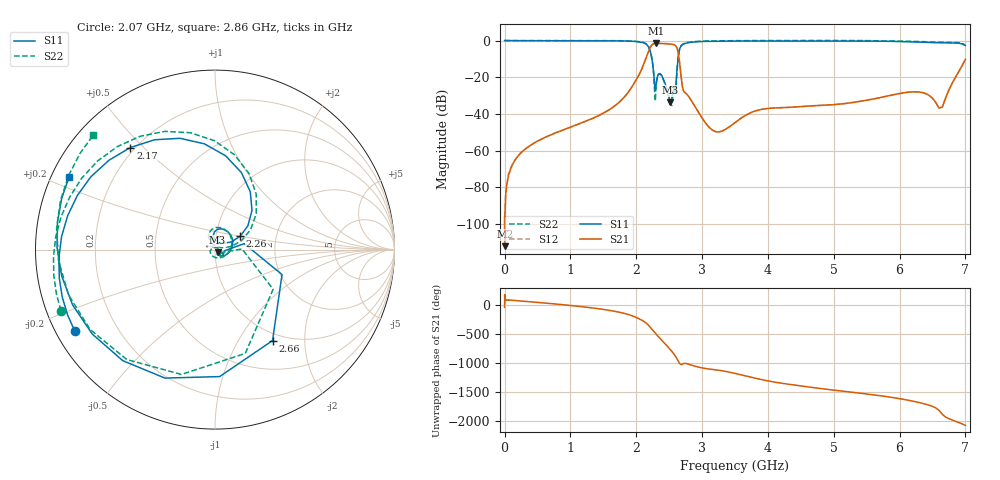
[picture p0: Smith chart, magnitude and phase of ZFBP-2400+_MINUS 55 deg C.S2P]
! Mini-Circuits
! S2P DATA File Format
! Type: BAND PASS FILTER
! Model: ZFBP-2400+
! All S Parameters are in dB deg format
! TEST CONDITIONS: INPUT POWER = 0 dBm @ Temperature = - 55 deg C
! 401 Frequency points
# MHz S DB R 50
!FREQMAG(S11)PHS(S11)MAG(S21)PHS(S21)MAG(S12)PHS(S12)MAG(S22)PHS(S22)
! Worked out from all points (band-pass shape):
!   401 points, 500 kHz to 7 GHz, reference 50 ohm
!   highest |S21| = -1.50 dB at 2.3 GHz (marker M1); lowest = -112.2 dB at 2 MHz (marker M2)
!   |S21| within 3 dB of the highest: 2.203 GHz to 2.623 GHz (420.7 MHz wide, 17.4 % of centre)
!   lowest |S11| = -33.6 dB at 2.52 GHz (marker M3), VSWR 1.04, Z = 51.4 - j1.55 ohm
!   |S11| at or under -10 dB: 2.238 GHz to 2.635 GHz (397 MHz wide, 16.3 % of centre)
!   |S22| runs from -35.5 to 0.1 dB; largest |S21 - S12| = 0.0011
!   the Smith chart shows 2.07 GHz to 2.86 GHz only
!   S11 on the Smith chart (normalised r, x): 2.07 GHz: 0.05, -0.27; 2.17 GHz: 0.18, +0.46; 2.26 GHz: 1.31, +0.20; 2.66 GHz: 0.89, -1.41; 2.86 GHz: 0.05, +0.23
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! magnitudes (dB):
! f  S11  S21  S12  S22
! 500 kHz  0.0  -96.1  -97.8  0.0
! 2 MHz  0.0  -112.2  -99.9  0.0
! 100 MHz  0.0  -69.5  -68.9  0.0
! 280 MHz  -0.1  -60.3  -60.1  0.0
! 1.17 GHz  -0.1  -44.9  -44.9  0.0
! 1.73 GHz  -0.2  -34.0  -34.0  0.0
! 2.07 GHz  -0.9  -16.7  -16.7  -0.7
! 2.17 GHz  -2.6  -7.4  -7.4  -2.4
! 2.26 GHz  -16.0  -1.8  -1.8  -16.2
! 2.3 GHz  -24.4  -1.5  -1.5  -25.8
! 2.34 GHz  -18.4  -1.5  -1.5  -18.2
! 2.52 GHz  -33.6  -1.9  -1.9  -34.7
! 2.56 GHz  -27.5  -2.1  -2.1  -29.3
! 2.66 GHz  -4.4  -12.5  -12.4  -4.4
! 2.74 GHz  -1.6  -28.4  -28.4  -1.4
! 2.86 GHz  -0.8  -34.1  -34.1  -0.6
! 3.18 GHz  -0.3  -49.3  -49.4  -0.1
! 3.52 GHz  -0.2  -44.2  -44.2  0.0
! 4.7 GHz  -0.2  -35.5  -35.5  0.1
! 5.85 GHz  -0.4  -30.0  -30.0  -0.2
! 6.6 GHz  -1.2  -36.9  -36.9  -0.8
! 7 GHz  -2.7  -10.2  -10.2  -2.4
